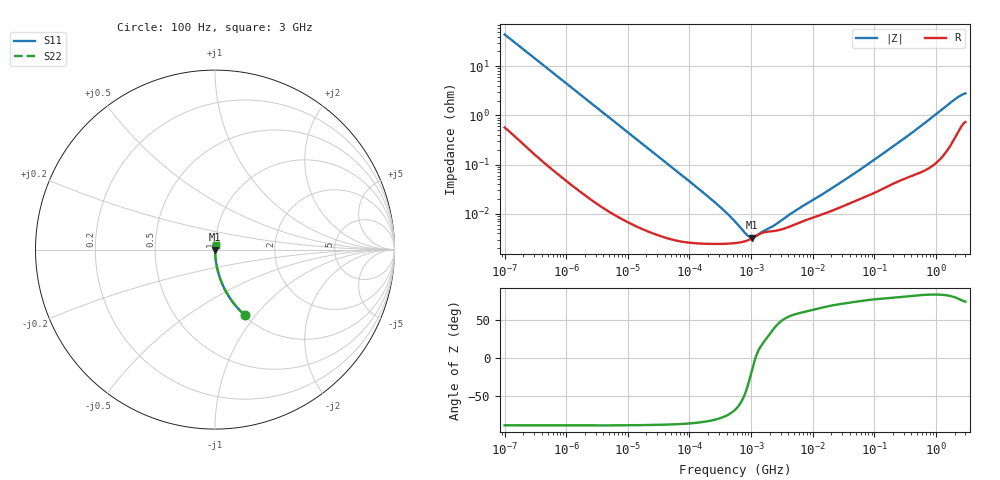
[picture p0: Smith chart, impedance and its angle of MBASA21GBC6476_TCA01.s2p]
! MBASA21GBC6476_TCA01  S-PARAMETER MODEL  ( Standard Model )
! Model Generated by TAIYO YUDEN Corporation (http://www.ty-top.com)
! Version 1.0
! TAIYO YUDEN Control No. 240524
! Copyright(c) 2024 TAIYO YUDEN CO.,LTD. All Rights Reserved.
! Product Description (link to TY-COMPAS)
! https://ds.yuden.co.jp/TYCOMPAS/or/detail?pn=MBASA21GBC6476MTCA01&u=M
! Products Name : Multilayer Ceramic Capacitors
! Characteristics :
!  Capacitance : 47 [uF] , Rated Voltage : 4 [V] , TCC : X6S
!  Case Size : 2.0 x 1.25 / 0.079 x 0.049 [mm/inch] , Thickness : 1.25 / 0.049 [mm/inch]
!  (Conditions: Temperature = 25 [degC] , DC Bias Voltage = 0 [V])
! External Node Assignments :
!  1  o---| |---o  2
! GND o---------o GND
! Frequency Range : 100Hz  -  3GHz  [ 401 STEP ]
# MHZ S RI R 50
! Freq[MHz].  S11 Real  S11 Imag  S21 Real  S21 Imag  S12 Real  S12 Imag  S22 Real  S22 Imag
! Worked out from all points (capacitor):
!   401 points, 100 Hz to 3 GHz, reference 50 ohm
!   read as one part in series: C = 36 uF near 109 Hz
!   lowest |Z| = 3.3 mohm at 1.045 MHz (marker M1)
!   series resonance near 1.177 MHz, so ESL is about 510 pH
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0.0001  0.1657 -0.3654  0.8343 0.3654  0.8343 0.3654  0.1657 -0.3654
0.000114  0.1338 -0.3341  0.8662 0.3341  0.8662 0.3341  0.1338 -0.3341
0.000175  0.0627 -0.2364  0.9373 0.2364  0.9373 0.2364  0.0627 -0.2364
0.000348  0.0174 -0.1253  0.9826 0.1253  0.9826 0.1253  0.0174 -0.1253
0.000724  0.00443 -0.0614  0.9956 0.0614  0.9956 0.0614  0.00443 -0.0614
0.001788  0.000896 -0.0251  0.9991 0.0251  0.9991 0.0251  0.000896 -0.0251
0.005476  0.000171 -0.00826  0.9998 0.00826  0.9998 0.00826  0.000171 -0.00826
0.031977  3.82e-05 -0.00143  1 0.00143  1 0.00143  3.82e-05 -0.00143
0.16412  2.49e-05 -0.000275  1 0.000275  1 0.000275  2.49e-05 -0.000275
0.388167  2.47e-05 -0.000105  1 0.000105  1 0.000105  2.47e-05 -0.000105
0.441669  2.49e-05 -8.92e-05  1 8.92e-05  1 8.92e-05  2.49e-05 -8.92e-05
0.547723  2.54e-05 -6.52e-05  1 6.52e-05  1 6.52e-05  2.54e-05 -6.52e-05
1.044606  3.19e-05 -8.3e-06  1 8.3e-06  1 8.3e-06  3.19e-05 -8.3e-06
4.141163  5.45e-05 7.83e-05  0.9999 -7.83e-05  0.9999 -7.83e-05  5.45e-05 7.83e-05
4.711951  5.81e-05 8.92e-05  0.9999 -8.92e-05  0.9999 -8.92e-05  5.81e-05 8.92e-05
9.794414  8.29e-05 0.000168  0.9999 -0.000168  0.9999 -0.000168  8.29e-05 0.000168
44.18008  0.000172 0.0006  0.9998 -0.0006  0.9998 -0.0006  0.000172 0.0006
175.1444  0.00038 0.00204  0.9996 -0.00204  0.9996 -0.00204  0.00038 0.00204
513.708  0.000689 0.00548  0.9993 -0.00548  0.9993 -0.00548  0.000689 0.00548
2036.508  0.00395 0.0209  0.996 -0.0209  0.996 -0.0209  0.00395 0.0209
2525.516  0.00629 0.0246  0.9937 -0.0246  0.9937 -0.0246  0.00629 0.0246
3000  0.008 0.0266  0.992 -0.0266  0.992 -0.0266  0.008 0.0266
